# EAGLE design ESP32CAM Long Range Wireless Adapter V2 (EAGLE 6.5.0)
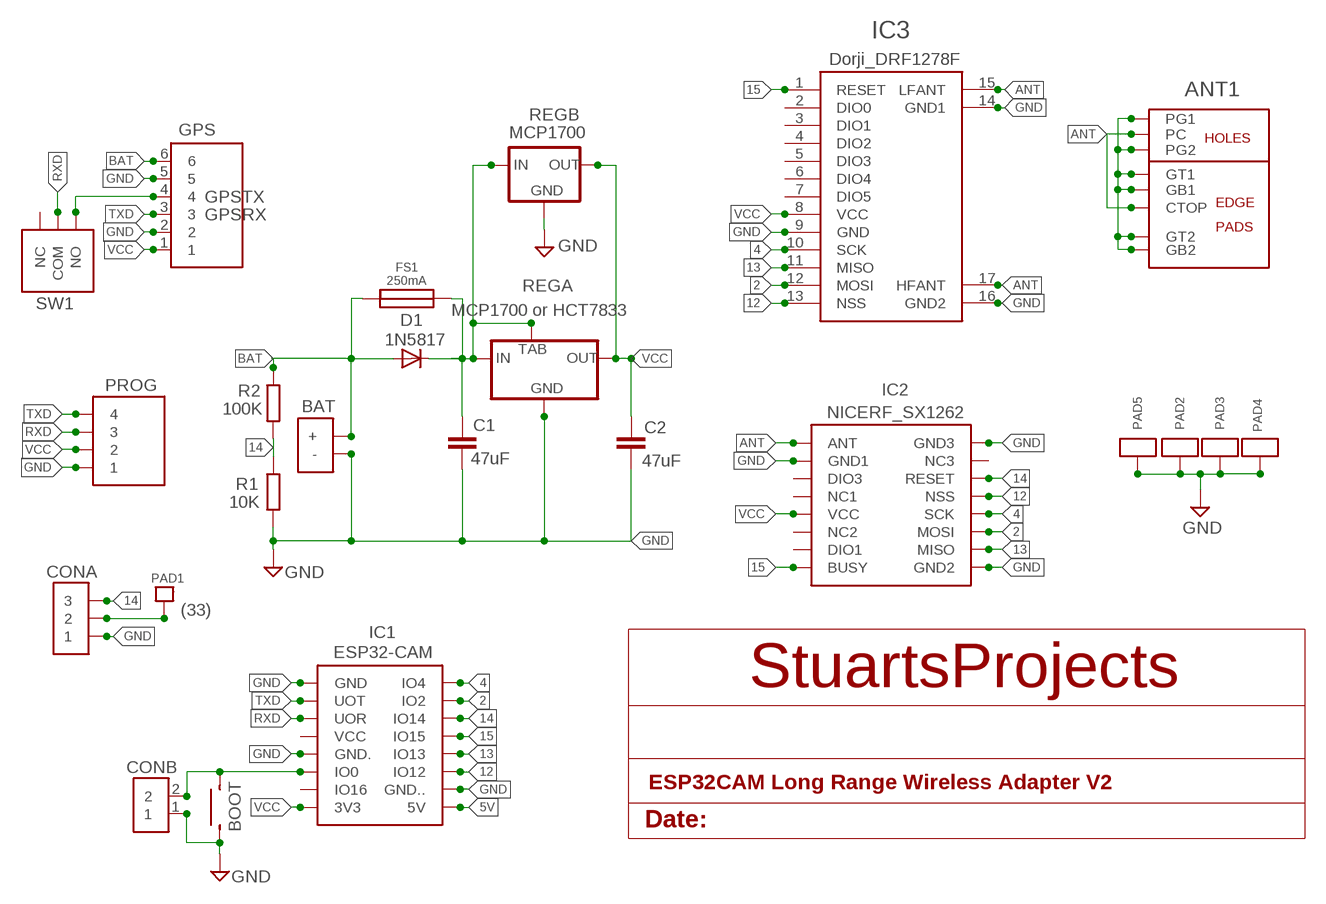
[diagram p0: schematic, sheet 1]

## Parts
ANT1  CUSTOMSMA  [CUSTOMSMA]
BAT  BATPADS2  [BATPADS]
BOOT  SMALLSMTSWITCH  [SMALLSMTSWITCH]
C1  47uF  C-EUC1206  [C1206]
C2  47uF  C-EUC1206  [C1206]
CONA  3X1  [3X1]
CONB  2X1  [2X1]
D1  1N5817  DIODE-DO41-7.6  [DO41-7.6]
FS1  250mA  SMALL_POLYFUSE  [SMALL_POLYFUSE]
GPS  6X1  [6X1]
IC1  ESP32-CAM  [ESP32-CAM]
IC2  NICERF_SX1262  [NICERF_SX1262]
IC3  Dorji_DRF1278F  DRF1278F_MULTI_SMT  [DRF1278F_MULTI_SMT]
PAD1  SINGLEPAD  [SINGLEPAD]
PAD2  ANTPAD2  [ANTPAD2]
PAD3  ANTPAD2  [ANTPAD2]
PAD4  ANTPAD2  [ANTPAD2]
PAD5  ANTPAD2  [ANTPAD2]
PROG  4X1  [4X1]
R1  10K  125MWRESISTORSTANDARD  [125MWRESISTOR]
R2  100K  125MWRESISTORSTANDARD  [125MWRESISTOR]
REGA  MCP1700 or HCT7833  MCP1700SOT89  [MCP1700SOT89]
REGB  MCP1700  [TO92REGB]
SW1  SMALL_PCB_SLIDE_DEFAULT  [SMALL_PCB_SLIDE]

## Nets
2: IC1.IO2 IC2.P$11(MOSI) IC3.12(MOSI)
4: IC1.IO4 IC2.P$12(SCK) IC3.10(SCK)
5V [POWER]: C1.1 D1.C FS1.P$2 IC1.5V REGA.2(IN) REGA.4(TAB) REGB.IN
12: IC1.IO12 IC2.P$13(NSS) IC3.13(NSS)
13: IC1.IO13 IC2.P$10(MISO) IC3.11(MISO)
14: CONA.3 IC1.IO14 IC2.P$14(RESET) R1.P$1 R2.P$2
15: IC1.IO15 IC2.P$8(BUSY) IC3.1(RESET)
ANT: ANT1.CTOP ANT1.PC IC2.P$1(ANT) IC3.15(LFANT) IC3.17(HFANT)
BAT [POWER]: BAT.BAT+(+) D1.A FS1.P$1 GPS.6 R2.P$1
GND [POWER]: ANT1.G1 ANT1.G2 ANT1.GB1 ANT1.GB2 ANT1.GT1 ANT1.GT2 BAT.BAT-V(-) BOOT.P$3 C1.2 C2.2 CONA.1 CONB.1 GPS.2 GPS.5 IC1.GND IC1.GND. IC1.GND.. IC2.P$2(GND1) IC2.P$9(GND2) IC2.P$16(GND3) IC3.9(GND) IC3.14(GND1) IC3.16(GND2) PAD2.P$1 PAD3.P$1 PAD4.P$1 PAD5.P$1 PROG.1 R1.P$2 REGA.1(GND) REGB.GND
N$1: BOOT.P$4 CONB.2 IC1.IO0
N$2: CONA.2 PAD1.P$1
N$3: GPS.4 SW1.NO
RXD: IC1.UOR PROG.3 SW1.COM
TXD: GPS.3 IC1.UOT PROG.4
VCC [VDD]: C2.1 GPS.1 IC1.3V3 IC2.P$5(VCC) IC3.8(VCC) PROG.2 REGA.3(OUT) REGB.OUT
Unconnected: IC1.IO16 IC1.VCC IC2.P$3(DIO3) IC2.P$4(NC1) IC2.P$6(NC2) IC2.P$7(DIO1) IC2.P$15(NC3) IC3.2(DIO0) IC3.3(DIO1) IC3.4(DIO2) IC3.5(DIO3) IC3.6(DIO4) IC3.7(DIO5) SW1.NC

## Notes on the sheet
- GPSTX
- GPSRX
- (33)

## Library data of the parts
ANT1 = con-coax:CUSTOMSMA
BAT = LMA2:BATPADS2
BOOT = LMA2:SMALLSMTSWITCH
C1 C2 = resistor:C-EU: CAPACITOR, European symbol
CONA = My_Pin_Headers:3X1
CONB = My_Pin_Headers:2X1
D1 = diode:DIODE-: DIODE
FS1 = LMA2:SMALL_POLYFUSE
GPS = My_Pin_Headers:6X1
IC1 = esp32:ESP32-CAM
IC2 = LMA2:NICERF_SX1262
IC3 = LMA2:DRF1278F_MULTI_SMT
PAD1 = LMA2:SINGLEPAD
PAD2-PAD5 = LMA2:ANTPAD2
PROG = My_Pin_Headers:4X1
R1 R2 = LMA2:125MWRESISTOR
REGA = LMA2:MCP1700SOT89
REGB = LMA2:MCP1700
SW1 = switch-tact:SMALL_PCB_SLIDE

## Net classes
0 default: width 0.254 mm
1 POWER: width 0.889 mm
2 VDD: width 0.889 mm
3 gpspower: width 0.889 mm

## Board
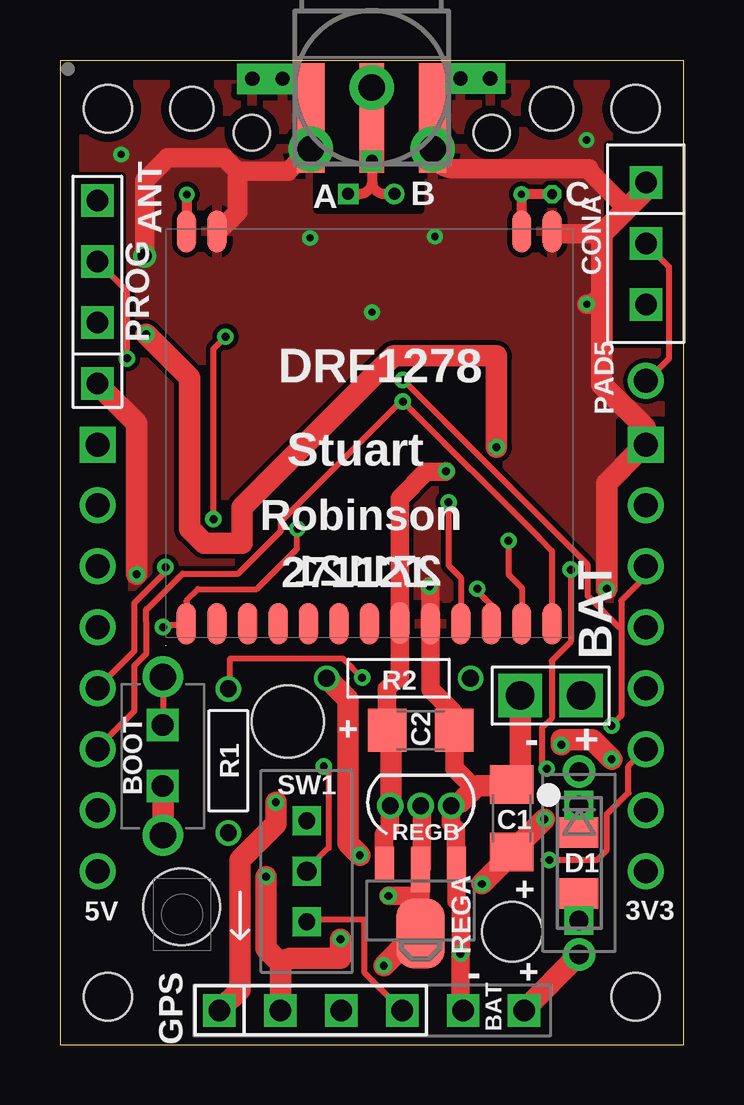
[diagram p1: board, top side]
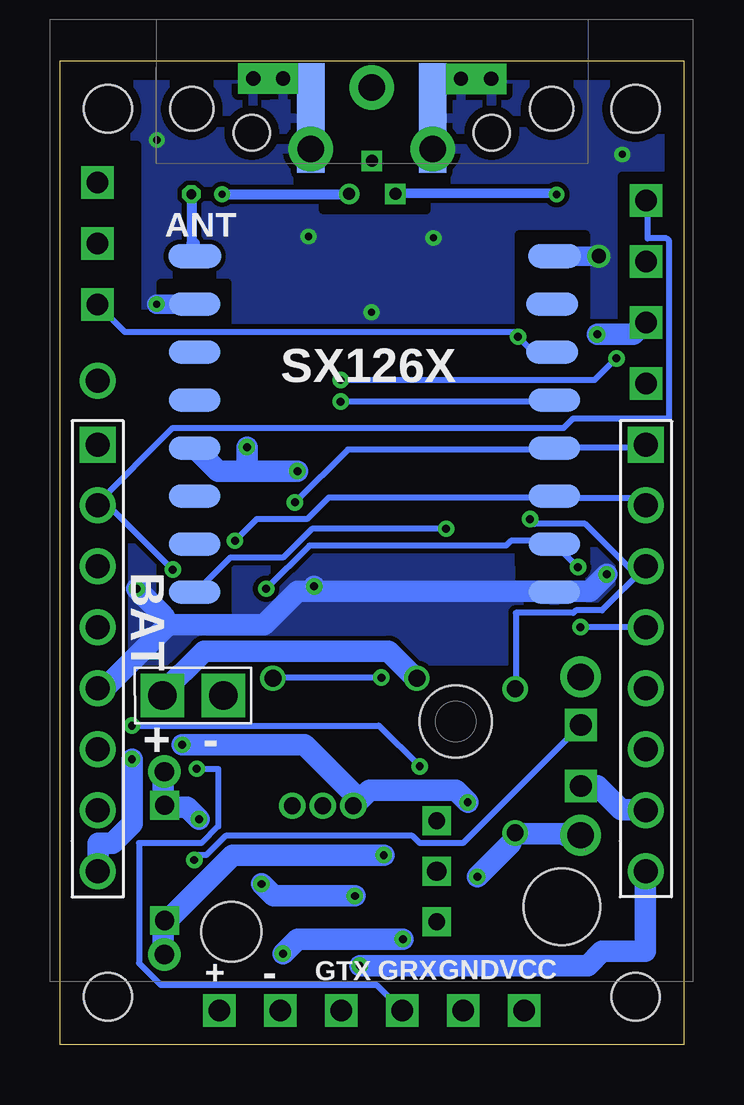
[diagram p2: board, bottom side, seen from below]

Size 26 x 41 mm. Coordinates in mm from the lower left corner, seen from the top.
Outline: 0,0 26,0 26,41 0,41 0,0
Copper layers (1*16): Top 0.0356mm / dielectric 1.5011mm / Bottom 0.0356mm
Design rules "LaenPCBOrder *": minimum track width 6mil, minimum drill 13mil, track to track 6mil, track to pad 6mil, pad to pad 6mil, via to via 6mil, smd to smd 6mil, copper to edge 15mil, drill to drill 6mil, minimum pad ring 7mil, minimum via ring 7mil, stop-mask expansion 3mil, vias tented up to drill 1000mil, thermal gap 10mil
Holes 3.2 mm at 5.07,5.75
Holes 1.5 mm at 8,38 18,38
Holes 3 mm at 9.5,13.47
Holes 2.5 mm at 18.85,4.71
Holes 2 mm at 2,2 24,2 2,39 24,39
Holes 1.8 mm at 5.5,39 20.5,39
tRestrict: area 0.5,26.5 to 2.6,36.2; area 22.9,29.2 to 26,37.5; area 5.6,0.3 to 20.4,2.5; area 0.5,6.2 to 2.6,26; area 23.4,6.2 to 25.5,26; area 11.1,35.8 to 15,40.9; area 10.7,34.8 to 15,36.3
bRestrict: area 23.4,6.2 to 25.5,26; area 22.8,29.3 to 26,37.5; area 0.6,26.6 to 2.6,36.2; area 0.5,6.2 to 2.6,26; area 4.1,20 to 6.8,33.8; area 19,18 to 21.8,31.7; area 11,35.9 to 15,41; area 9.9,36.3 to 11,36.3; area 15.2,36.3 to 15.9,36.3; area 5,19.4 to 6.8,20.1; area 22,30.4 to 22.6,30.4; area 10.7,34.8 to 15,36.3

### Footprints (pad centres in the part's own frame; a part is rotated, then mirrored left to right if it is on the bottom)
CUSTOMSMA = smd 4.572 x 1.016: CTOP -1.27,0 | drill 1.1 pad 1.85: G1 -2.55,2.55; G2 -2.55,-2.55; PC 0,0 | smd 4.572 x 1.143 bottom: GB1 -1.27,2.54; GB2 -1.27,-2.54 | smd 4.572 x 1.143: GT1 -1.27,2.54; GT2 -1.27,-2.54
BATPADS = drill 1.2 pad 1.778 square: BAT+ 0,-1.27; BAT-V 0,1.27
SMALLSMTSWITCH = drill 1.1 pad 1.7: P$3 -3.3,0; P$4 3.3,0
C1206 = smd 1.6 x 1.8: 1 -1.4,0; 2 1.4,0
3X1 = drill 0.9 square: 1 -2.54,0; 2 0,0; 3 2.54,0
2X1 = drill 0.9 square: 1 -1.27,0; 2 1.27,0
DO41-7.6 = drill 0.8 pad 1.35: A 3.81,0; C -3.81,0
SMALL_POLYFUSE = drill 0.8 square: P$1 -2.4,0; P$2 2.4,0 | smd 1.27 x 1.635: P$3 -1.27,0; P$4 1.27,0
6X1 = drill 0.9 square: 1 -6.35,0; 2 -3.81,0; 3 -1.27,0; 4 1.27,0; 5 3.81,0; 6 6.35,0
ESP32-CAM = drill 1: 3V3 -11.43,3.81; 5V 11.43,3.81; GND. -11.43,11.43; GND.. 11.43,6.35; IO0 -11.43,8.89; IO2 11.43,19.05; IO12 11.43,8.89; IO13 11.43,11.43; IO14 11.43,16.51; IO15 11.43,13.97; IO16 -11.43,6.35; UOR -11.43,16.51; UOT -11.43,19.05; VCC -11.43,13.97 | drill 1 square: GND -11.43,21.59; IO4 11.43,21.59
NICERF_SX1262 = smd 2.2 x 1: P$1 -7.5,7.5; P$16 7.5,7.5 | smd 2.159 x 0.965: P$2 -7.5,5.5; P$3 -7.5,3.5; P$4 -7.5,1.5; P$5 -7.5,-0.5; P$6 -7.5,-2.5; P$7 -7.5,-4.5; P$8 -7.5,-6.5; P$9 7.5,-6.5; P$10 7.5,-4.5; P$11 7.5,-2.5; P$12 7.5,-0.5; P$13 7.5,1.5; P$14 7.4,3.5; P$15 7.4,5.5
DRF1278F_MULTI_SMT = smd 0.8 x 1.75: 1 16.13,16.45; 2 14.85,16.45; 3 13.57,16.45; 4 12.3,16.45; 5 11.04,16.45; 6 9.77,16.45; 7 8.5,16.45; 8 7.23,16.42; 9 5.96,16.45; 10 4.69,16.45; 11 3.42,16.45; 12 2.15,16.45; 13 0.88,16.45; 14 14.85,0.1; 15 16.12,0.1; 16 0.88,0.1; 17 2.15,0.1
SINGLEPAD = drill 1: P$1 0,0
ANTPAD2 = drill 0.6 pad 1.27 square: P$1 0,0
4X1 = drill 0.9 square: 1 -3.81,0; 2 -1.27,0; 3 1.27,0; 4 3.81,0
125MWRESISTOR = drill 0.7: P$1 -3,0; P$2 3,0
MCP1700SOT89 = smd 0.8 x 1.4: 1 -1.499,-1.981; 3 1.499,-1.981 | smd 0.8 x 1.9: 2 0,-1.727 | smd 2.032 x 2.921: 4 0,0.94
TO92REGB = drill 0.7 pad 1.1: GND -1.27,-1.2; IN 0,-1.2; OUT 1.27,-1.2
SMALL_PCB_SLIDE = drill 0.8 pad 1.2 square: COM 0,0 | drill 0.7 pad 1.2 square: NC 2.1,0; NO -2.1,0

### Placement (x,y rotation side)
ANT1  13,39.88 90 top
BAT  20.46,14.55 90 top
BOOT  4.29,12.03 90 top
C1  18.83,9.44 90 top
C2  15.04,13.1 0 top
CONA  24.43,33.38 270 top
CONB  4.28,12.05 90 top
D1  21.65,7.57 270 top
FS1  21.64,7.58 90 top
GPS  13,1.43 0 top
IC1  13,3.42 0 bottom
IC2  12.88,25.36 0 bottom
IC3  21.4,33.99 180 top
PAD1  24.43,27.66 0 top
PAD2  17.94,40.26 0 top
PAD3  8.02,40.25 0 top
PAD4  9.28,40.25 0 top
PAD5  16.7,40.26 0 top
PROG  1.56,31.37 90 top
R1  7.02,11.83 270 top
R2  14.12,15.27 0 top
REGA  15.03,5.58 180 top
REGB  15.04,8.76 180 top
SW1  10.29,7.23 90 top

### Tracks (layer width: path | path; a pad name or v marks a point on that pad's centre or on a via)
2  (via drill 0.33)
  Top 0.254: 19.2,17.6 IC3.12 19.25,19.05 18.7,19.6 v18.7,21
  Bottom 0.254: v18.7,21 17.8,21.9 15.7,21.9 14.8,22.8 5.4,22.8 IC2.P$11 5.3,22.8 1.9,22.8 1.6,22.5 IC1.IO2
4  (via drill 0.33)
  Top 0.254: 16.7,17.6 IC3.10 16.71,19.46 16.2,19.97 v16.2,22.6
  Bottom 0.254: v16.2,22.6 14,24.8 5.4,24.8 IC2.P$12 5.3,24.9 1.7,24.9 1.6,25 IC1.IO4
5V  (via drill 0.33)
  Top 0.762: 15.1,9.9 15.1,7.38 REGA.2 15.03,6.3 | 15.03,6.3 REGA.4 | v13.7,6.2 14.93,6.2 15.03,6.3
  Top 0.889: v20.2,9.4 18.9,8.1 C1.1 18.6,7.7 v17.6,6.7 | 15.1,9.9 REGB.IN | 15.1,4.7 REGA.4 14.6,4.5 14.6,4.4 v13.5,3.3
  Bottom 0.889: v20.2,9.4 20.7,9.9 21.6,9.9 FS1.P$2 21.7,10.4 21.7,11.3 D1.C | v13.5,3.3 4,3.3 3.4,3.9 1.6,3.9 1.6,7.2 IC1.5V | v17.6,6.7 17.1,6.2 v13.7,6.2
12  (via drill 0.33)
  Top 0.254: 20.5,17.6 IC3.13 20.51,20.59 20,21.1 v14.3,26.8 14.2,26.8 9.2,21.8 9.2,21.4 7.43,19.63 5.12,19.63 4.93,19.44 4.92,19.44 3.63,18.15 3.6,18.15 3.6,17.6 3.6,16.3 3.1,15.8 3.1,13.9 1.6,12.4 IC1.IO12
  Bottom 0.254: v14.3,26.8 5.4,26.8 IC2.P$13
13  (via drill 0.33)
  Top 0.254: 17.9,17.6 IC3.11 17.98,18.31 17.4,18.89 v17.4,19 | v4.4,19.9 4.4,19.7 3.1,18.4 3.1,16.4 1.6,14.9 IC1.IO13
  Bottom 0.254: v17.4,19 15.6,20.8 7.4,20.8 7.2,21 5.5,21 5.4,20.9 IC2.P$10 5.3,20.8 v4.4,19.9
14  (via drill 0.33)
  Top 0.254: v12.6,15.3 11.8,16.1 7.1,16.1 7.1,14.9 R1.P$1 | v6.9,29.5 6.4,29 v6.4,21.9
  Bottom 0.254: IC2.P$14 5.5,28.9 6.3,28.9 v6.9,29.5 6.9,29.6 6.9,29.7 23.3,29.7 24.4,30.8 CONA.3 | R1.P$1 7,14.9 7,18 4.6,18 4.5,18.1 3.4,18.1 1.6,19.9 IC1.IO14 2,19.6 4.1,21.7 6.2,21.7 v6.4,21.9 | v12.6,15.3 17.1,15.3 R2.P$2
15  (via drill 0.33)
  Top 0.254: v4.3,17.4 4.3,17.5 5.2,17.5 IC3.1 5.3,17.6 5.3,18.43 5.29,18.44 5.29,18.52 5.75,18.98 8.19,18.98 9.88,20.67 9.88,21.48 v9.9,21.5
  Bottom 0.254: v4.3,17.4 1.6,17.4 IC1.IO15 | v9.9,21.5 15.5,21.5 16.7,20.3 18.9,20.3 20.3,18.9 IC2.P$8
ANT  (via drill 0.3, 0.4, 0.5)
  Top 0.254: ANT1.PC 13,39.8 13,38.8 ANT1.CTOP | v13,36.83 13.03,36.83
  Top 0.406: IC3.15 5.31,35.28 v5.29,35.43 | 13.03,35.86 13.03,36.36 | 13.03,36.36 13.03,36.83 | 13.03,36.83 13.03,37.01 | 13.03,37.01 13,37.64 | 13,37.64 ANT1.CTOP | 13.03,35.93 13.03,36.36 | 13.03,36.36 13.03,36.83 | 13.03,36.83 13.03,37.01 | 13.03,37.01 13,37.64 | IC3.17 v19.24,35.44 v20.52,35.44 | v12.02,35.45 arc90 v12.03,35.44 12.45,35.44 arc90 13.03,36.02 13.03,36.36 | v13.94,35.45 13.52,35.45 arc-90 13.03,35.94 13.03,36.36
  Bottom 0.254: 5.49,35.47 5.33,35.47 v5.29,35.43
  Bottom 0.406: 5.49,35.47 v12.02,35.45 | 20.22,32.89 arc-90 20.25,32.86 20.31,32.86 IC2.P$1 20.38,33.4 20.52,33.4 v20.52,35.44 | 20.22,32.89 20.41,32.89 | v19.24,35.44 13.93,35.43 v13.94,35.45 | 20.22,32.89 20.39,32.89 | v20.52,35.44 20.5,35.44 v20.52,35.44
BAT  (via drill 0.33)
  Top 0.889: GPS.6 19.4,1.5 21.6,3.7 D1.A | v12.5,7.9 12,8.4 12,14.4 11.2,15.2 R2.P$1
  Bottom 0.889: D1.A 21.7,3.8 21.7,5.1 FS1.P$1 21.3,5.4 18.8,7.9 v12.5,7.9 | R2.P$1 11.2,15.3 12.3,16.4 20,16.4 21.8,14.6 BAT.BAT+
GND  (via drill 0.3, 0.33, 0.6)
  Top 0.762: 16.4,13.1 16.4,13.85 15.44,14.81 IC3.9 15.44,19.06 v15.4,19.1 | 16.3,9.9 16.3,9.22 16.51,9.01 16.51,7.58 REGA.1 16.53,6.15 16.53,6.01 16.71,5.83 v16.71,3.81 v16.7,3.8 16.7,1.54 GPS.5 | C2.2 16.44,11.52 17.28,10.68 | PAD2.P$1 PAD5.P$1 15.56,40.26 15.55,40.27 ANT1.GT2 | PAD3.P$1 PAD4.P$1 10.44,40.25 10.47,40.22 ANT1.GB1
  Top 0.813: v21.97,30.86 arc90 22.6,31.49 22.6,31.64 | IC3.16 arc90 20.61,33.8 22.6,33.8 | ANT1.G2 arc90 16.37,36.51 22.06,36.51 22.06,36.41 23.64,34.84 | v3.53,32.86 3.53,36 4.48,36.95 6.85,36.95 7.4,36.4 | 7.4,36.4 9.52,36.4 ANT1.G1 | IC3.14 6.6,33.89 7.4,34.69 7.4,36.4
  Top 0.889: ANT1.G2 15.5,37.4 15.5,38.2 ANT1.GT2 | ANT1.G1 10.5,37.4 10.5,38.2 ANT1.GB1 | 9.2,3.4 9.2,1.5 GPS.2 | 9.2,3.4 8.6,4 v8.6,7 | CONB.1 4.3,10.7 4.3,8.8 BOOT.P$3 | 16.4,13.1 C2.2 | 16.3,9.9 REGB.GND 16.7,10.1 17.28,10.68 17.4,10.8 18.8,10.8 C1.2 19.2,11.1 19.2,14.5 BAT.BAT-V | v11.7,4.4 11.7,3.6 9.6,3.6 9.2,3.4 | CONA.1 24.4,35.9 24.4,35.6 23.64,34.84 22.6,33.8 22.6,31.64 22.6,27.5 24.4,25.7 24.4,25.1 IC1.GND 24.1,24.7 22.8,23.4 v22.8,19 | v3.2,19.6 3.2,25.9 1.6,27.5 PROG.1
  Bottom 0.813: IC2.P$2 v21.97,30.86 | IC2.P$16 v3.53,32.86
  Bottom 0.889: ANT1.GT2 15.5,38.6 15.5,37.4 ANT1.G2 15.1,37.3 | ANT1.GB1 10.5,38.6 10.5,37.4 ANT1.G1 10.9,37.3 | BOOT.P$3 4.3,8.7 4.9,8.7 5,8.8 7,8.8 R1.P$2 7.2,8.4 v8.6,7 | IC1.GND.. 1.6,9.8 2.6,9.8 3.6,10.8 4.2,10.8 CONB.1 | v11.7,4.4 16.1,4.4 v16.7,3.8 | 15.4,18.9 16.1,18.9 17.5,17.5 21.5,17.5 | 15.4,18.9 5.4,18.9 IC2.P$9 5,18.9 3.9,18.9 v3.2,19.6 | 21.5,17.5 24.1,14.9 24.4,14.9 IC1.GND. | v22.8,19 21.7,17.9 21.5,17.5 | v15.4,19.1 15.4,18.9
  other vias: 13.01,30.52 15.64,33.68 10.43,33.62 2.55,37.1 21.96,37.7
  pour Top (isolate 0.2): 1,40 25,40 25,17 1,17
  pour Bottom (isolate 0.2): 1,40 25,40 25,16 1,16
N$1  (via drill 0.33)
  Top 0.254: CONB.2 4.3,13.4 4.3,15.3 BOOT.P$4 | v20.4,7.7 22.4,7.7 22.8,8.1 22.8,9.6 23.7,10.5 23.7,11.6 24.4,12.3 IC1.IO0
  Bottom 0.254: v20.4,7.7 20.2,7.9 19.9,7.9 19.1,8.7 11.3,8.7 11,8.4 9.2,8.4 4.3,13.3 CONB.2
N$2
  Top 0.254: CONA.2 24.5,33.3 25.4,32.4 25.4,28.6 24.5,27.7 PAD1.P$1
N$3
  Top 0.254: SW1.NO 10.3,5.2 12.7,5.2 12.7,3 14.2,1.5 GPS.4
RXD  (via drill 0.33)
  Top 0.254: v11,11.6 11.2,11.4 11.2,8.2 10.3,7.3 SW1.COM | v23,13.3 23.4,13.7 23.4,17.4 | 23.4,17.4 23.4,18.5 24.4,19.5 24.4,19.9 IC1.UOR | v2.8,28.6 2.8,31.4 1.6,32.6 PROG.3 | v14.3,27.7 22,20 22,18.7 23.3,17.4 23.4,17.4
  Bottom 0.254: v11,11.6 12.7,13.3 v23,13.3 | v2.8,28.6 3.7,27.7 v14.3,27.7
TXD  (via drill 0.33)
  Top 0.254: v20.3,11.5 20.1,11.7 20.1,13.2 20.5,13.6 20.5,16 21.3,16.8 v21.3,19.8
  Bottom 0.254: v20.3,11.5 19.4,11.5 19.4,9.1 20.1,8.4 22.7,8.4 22.7,3.4 21.8,2.5 12.8,2.5 11.8,1.5 GPS.3 | v21.3,19.8 23.9,22.4 24.4,22.4 IC1.UOT 24.5,22.5 21.3,25.7 5,25.7 4.6,26.1 0.6,26.1 0.6,33.5 0.7,33.6 1.5,33.6 1.5,35.1 PROG.4
VCC  (via drill 0.33)
  Top 0.762: v16.1,23.9 16.07,23.87 15.26,23.87 14.17,22.78 IC3.8 14.17,15.36 13.64,14.83 C2.1 | REGB.OUT 13.77,9.03 13.52,8.78 13.52,7.57 REGA.3
  Top 0.889: v9,10.1 9,9.2 7.5,7.7 7.5,2.3 6.7,1.5 GPS.1 | v23,11.9 22.2,12.7 20.9,12.7 v20.9,12.5 | 13.9,13.3 13.7,13.1 C2.1 13.8,12.7 13.8,10.4 REGB.OUT | v3.6,29.6 5.4,27.8 5.4,21.5 6,20.9 7.6,20.9 7.6,22.4 13.9,28.7 18.2,28.7 v18.2,24.9
  Bottom 0.889: v9,10.1 9.5,10.6 13.1,10.6 13.7,10 REGB.OUT 13.8,10.5 15.8,12.5 v20.9,12.5 | v23,11.9 23,9.2 23.8,8.4 24.4,8.4 24.4,7.3 IC1.3V3 | v16.1,23.9 18.2,23.9 | 18.2,23.9 19.4,23.9 20.3,24.8 IC2.P$5 | v3.6,29.6 2.1,29.6 1.6,30.1 PROG.2 | v18.2,24.9 18.2,24.3 18.2,23.9

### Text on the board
tPlace: A | B | C
tNames: ANT | CONA | PROG | DRF1278 | PAD5 | Stuart | Robinson | 271121 | 271121 | R2 | BAT | BOOT | + | - | + | C2 | R1 | SW1 | REGB | C1 | + | D1 | 5V | 3V3 | REGA | - | + | GPS | BAT
bNames: ANT | SX126X | BAT | - | + | - | + | VCC | GND | GRX | GTX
